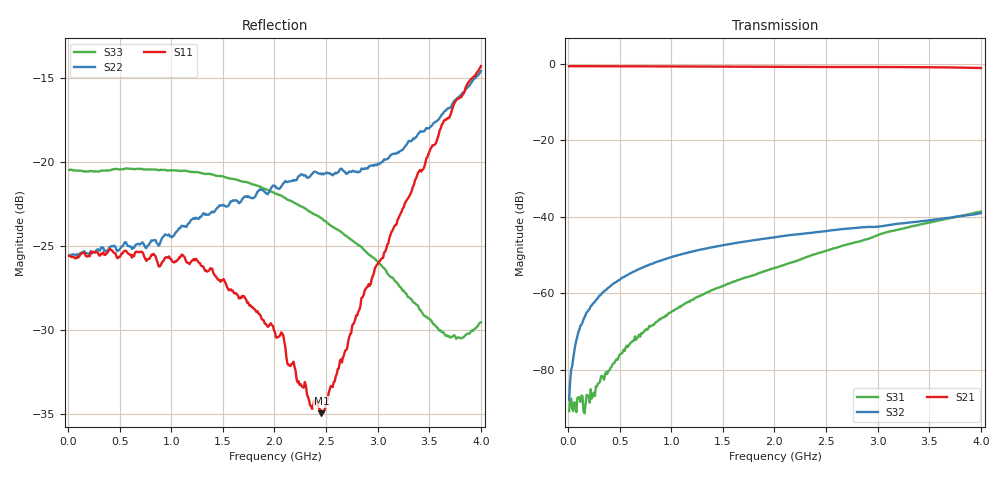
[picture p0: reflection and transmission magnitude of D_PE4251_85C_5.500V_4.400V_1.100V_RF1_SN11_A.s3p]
! Device ID: PE4251_SoldCshunt_081809
! Dir: c:\Test Bench Repositories\Bench_Software_CVI_Version_8\trunk\PSC 4Port_VNA Bench\datalog\4250\TEST\PE4251_SoldCshunt_081809\85C\5p500000\RF1
! Serial: 11
! Insertion: A
! Temp: 85C
! VDD: 5.500
! Control_Hi: 80.000
! Control_Lo: 20.000
! Logic State: RF1
! Port 1: RFC
! Port 2: RF1
! Port 3: RF2
! V1 = 1.10
! V2 = 4.40
! V3 = 1.10
! IDD: 6.786960e-05
! FILE NAME
! DATE 08/18/09  20:19
! CORRECTED  DATA
#  Hz  S  RI  R  50.00
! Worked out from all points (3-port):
!   401 points, 10 MHz to 4 GHz, reference 50 ohm
!   strongest paths, dB at 10 MHz, 1.008 GHz, 2.005 GHz, 3.002 GHz, 4 GHz:
!     S21: -0.6, -0.7, -0.8, -0.8, -1.1
!     S32: -87.8, -50.5, -45.3, -42.6, -39.0
!     S31: -90.8, -64.7, -53.3, -44.7, -38.6
!   lowest |S11| = -35.0 dB at 2.454 GHz (marker M1), VSWR 1.04, Z = 49.9 - j1.79 ohm
!   |S11| at or under -10 dB: start of sweep to end of sweep
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1e7  0.0526 0.000126  0.9312 -0.00338  7.37e-05 -2.28e-05
     0.9304 -0.00518  0.0529 0.000153  5.43e-05 0.000118
     -9.44e-06 -2.73e-05  2.02e-05 -3.55e-05  0.0947 -0.000184
9.9775e7  0.052 -0.00108  0.9327 -0.0347  3.85e-05 -2.58e-05
          0.9317 -0.0351  0.0528 -0.000962  5.11e-05 0.000301
          3.09e-05 -3.14e-05  3.94e-05 0.000311  0.0944 -0.00206
1.79575e8  0.0523 -0.00118  0.9292 -0.0617  6.1e-06 -3.87e-05
           0.9289 -0.0619  0.0535 -0.00112  6.11e-05 0.00054
           1.2e-05 -4.56e-05  5.57e-05 0.000561  0.0937 -0.00415
3.8905e8  0.0541 -0.00412  0.9212 -0.1308  -6.83e-05 -7.18e-05
          0.9208 -0.1302  0.0545 -0.00322  0.000107 0.00118
          -6.35e-05 -7.24e-05  0.000107 0.00117  0.094 -0.0102
5.18725e8  0.0531 -0.00595  0.9123 -0.1726  -0.000133 -8.58e-05
           0.9125 -0.1727  0.0559 -0.00451  0.000154 0.00156
           -0.000138 -8.86e-05  0.000138 0.00158  0.0943 -0.0129
1.1671e9  0.0474 -0.016  0.8441 -0.3737  -0.000774 -6.88e-05
          0.8444 -0.3735  0.063 -0.0188  0.000573 0.00337
          -0.000778 -7.66e-05  0.000559 0.00338  0.0907 -0.0239
2.005e9  0.0255 -0.0178  0.7015 -0.584  -0.00216 0.000157
         0.7014 -0.5837  0.0716 -0.0459  0.000985 0.00533
         -0.00216 0.000142  0.000981 0.00532  0.0748 -0.0303
2.453875e9  -0.000447 -0.0179  0.6085 -0.6749  -0.00342 0.000243
            0.6073 -0.6759  0.0612 -0.0686  0.00106 0.00631
            -0.00343 0.000249  0.00105 0.00633  0.0603 -0.0316
3.66085e9  -0.1125 -0.0719  0.2758 -0.857  -0.00892 0.00284
           0.2787 -0.8553  -0.0631 -0.1276  -0.000137 0.0096
           -0.00896 0.00279  -0.000133 0.00963  0.0048 -0.03
4e9  -0.1765 -0.0782  0.1545 -0.8729  -0.0109 0.00443
     0.1541 -0.8701  -0.1371 -0.1265  -0.000728 0.0111
     -0.0109 0.00436  -0.000761 0.0111  -0.0155 -0.0296
